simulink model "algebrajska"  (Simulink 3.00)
settings: Solver=ode4  StartTime=0.0  StopTime=10  FixedStep=0.0001  RelTol=1e-3

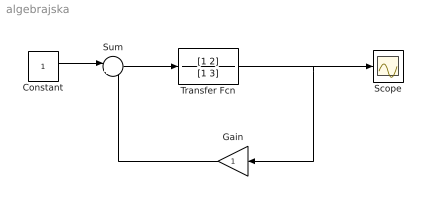
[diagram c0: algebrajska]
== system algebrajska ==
  Constant : Constant  Value=1
  Gain : Gain  Orientation=left  Gain=1  SaturateOnIntegerOverflow=on
  Scope : Scope
  Sum : Sum  Inputs=|+-  SaturateOnIntegerOverflow=on
  Transfer Fcn : TransferFcn  Numerator=[1 2]  Denominator=[1 3]
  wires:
  Constant/1 -> Sum/1
  Sum/1 -> Transfer Fcn/1
  Transfer Fcn/1 -> Scope/1, Gain/1
  Gain/1 -> Sum/2
